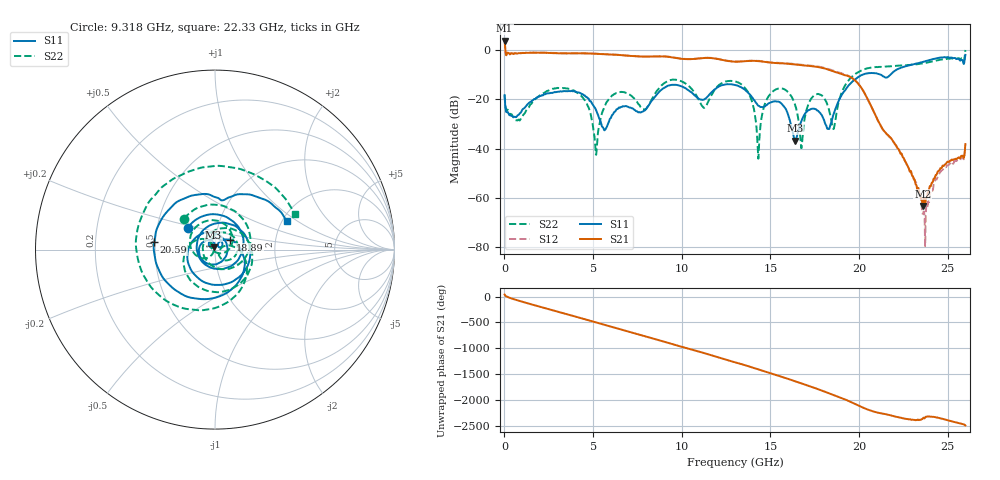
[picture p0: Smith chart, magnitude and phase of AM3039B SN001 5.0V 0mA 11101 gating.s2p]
!Agilent Technologies,E8364B,MY43040894,A.07.50.67
!Agilent E8364B: A.07.50.67
!Date: Tuesday, June 28, 2016 08:13:02
!Correction: S11(Full 2 Port(1,2))
!S21(Full 2 Port(1,2))
!S12(Full 2 Port(1,2))
!S22(Full 2 Port(1,2))
!S2P File: Measurements: S11, S21, S12, S22:
# Hz S  dB  R 50
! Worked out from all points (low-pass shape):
!   1601 points, 10 MHz to 26 GHz, reference 50 ohm
!   highest |S21| = 3.88 dB at 10 MHz (marker M1); lowest = -63.3 dB at 23.6 GHz (marker M2)
!   |S21| within 3 dB of the highest: start of sweep to 43.86 MHz
!   lowest |S11| = -36.8 dB at 16.38 GHz (marker M3), VSWR 1.03, Z = 49.2 + j1.21 ohm
!   |S11| at or under -10 dB: start of sweep to 20.19 GHz; 21.23 GHz to 21.77 GHz (538.7 MHz wide, 2.51 % of centre)
!   |S22| runs from -44.1 to 0.1 dB; largest |S21 - S12| = 0.024
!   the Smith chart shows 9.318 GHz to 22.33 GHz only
!   S11 on the Smith chart (normalised r, x): 9.318 GHz: 0.72, +0.18; 18.89 GHz: 1.17, +0.13; 20.59 GHz: 0.49, +0.05; 22.33 GHz: 2.12, +0.84
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1e7  -18.29 54.7  3.88 41.0  3.94 41.8  -18.37 22.4
7.734562e8  -26.41 43.2  -1.24 -74.4  -1.18 -74.2  -28.33 -6.9
1.780569e9  -19.52 -34.2  -1.03 -174.3  -0.97 -174.0  -19.66 -58.9
2.885144e9  -17.07 -172.8  -1.23 79.8  -1.17 80.2  -15.54 173.5
4.347081e9  -17.84 0.2  -1.29 -58.9  -1.26 -58.6  -18.74 -2.4
5.484144e9  -30.60 -103.9  -1.60 -169.8  -1.54 -169.3  -26.00 16.4
6.491256e9  -23.34 -125.1  -1.98 92.0  -1.90 92.6  -17.09 -103.1
7.514612e9  -25.05 86.9  -2.56 -6.4  -2.50 -5.9  -21.51 109.0
8.684162e9  -17.27 -130.0  -2.49 -119.5  -2.43 -118.9  -15.84 -136.9
9.317669e9  -14.23 141.0  -2.77 175.5  -2.69 175.9  -12.24 135.3
1.113697e10  -20.17 -143.2  -3.26 0.1  -3.21 0.6  -22.59 -133.0
1.3005e10  -14.13 -91.3  -4.71 168.7  -4.64 169.1  -12.70 -104.5
1.45644e10  -23.15 -17.1  -4.65 3.9  -4.54 4.6  -25.11 -129.3
1.63837e10  -36.76 122.3  -5.80 163.4  -5.65 164.2  -22.02 2.4
1.734208e10  -23.81 88.0  -6.51 50.9  -6.34 52.1  -19.35 63.1
1.888524e10  -20.00 33.3  -9.38 -147.1  -9.10 -145.9  -20.22 11.3
2.059083e10  -9.35 173.1  -21.34 -39.9  -21.42 -39.9  -7.18 -178.9
2.167916e10  -10.60 76.6  -34.89 -129.9  -34.97 -131.5  -6.62 78.6
2.232891e10  -7.28 21.8  -41.90 174.5  -41.50 170.4  -6.24 23.7
2.359592e10  -4.77 -85.5  -63.27 158.5  -66.44 125.3  -5.34 -75.5
2.483045e10  -2.87 167.9  -46.50 142.0  -47.47 141.2  -3.56 -174.1
2.6e10  -1.91 25.0  -38.17 24.8  -38.43 20.5  0.07 57.6
